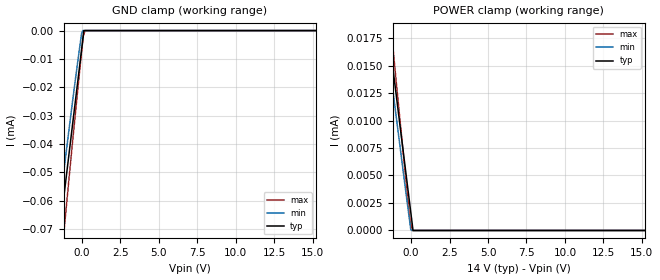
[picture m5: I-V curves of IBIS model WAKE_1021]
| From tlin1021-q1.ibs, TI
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|   WAKE
[Model]   WAKE_1021
Model_type   Input
Vinl = 11
Vinh = 12
|   typ   min   max
C_comp   3.243pF   2.436pF   4.514pF
[Voltage Range]   14   4.5   36
[Temperature Range]   25   165   -55
[Power Clamp Reference]   14   4.5   36
[GND Clamp Reference]   0   0   0
[GND Clamp]
|   Voltage   I(typ)   I(min)   I(max)
-14V      -714.2uA   -631.4uA   -824.8uA
-2.002V   -97.93uA   -85.92uA   -118.4uA
-1.479V   -72.07uA   -62.72uA   -88.41uA
-1.419V   -69.35uA   -60.05uA   -84.94uA
-1.039V   -52.29uA   -43.4uA    -63.3uA
-199.5mV  -14.56uA   -7.89uA    -16.73uA
-19.59mV  -6.478uA   -864.9nA   -7.077uA
56.56mV   -3.056uA   0A         -3.029uA
76.07mV   -2.18uA    0A         -1.992uA
124.6mV   0A         0A         -1.235uA
203.6mV   0A         0A         0A
36V       0A         0A         0A
[POWER Clamp]
|   Voltage   I(typ)   I(min)   I(max)
-14V      176.2uA    156.4uA    203.4uA
-2.462V   30.39uA    26.89uA    35.18uA
-1.479V   18.07uA    15.98uA    20.93uA
-1.419V   17.39uA    15.32uA    20.05uA
-1.176V   14.66uA    12.64uA    16.55uA
-618.9mV  8.378uA    6.516uA    8.546uA
-77.33mV  2.275uA    661.2nA    927.9nA
-19.59mV  1.625uA    44.14nA    578.6nA
56.56mV   766.5nA    0A         118nA
76.07mV   546.7nA    0A         0A
124.6mV   0A         0A         0A
36V       0A         0A         0A
